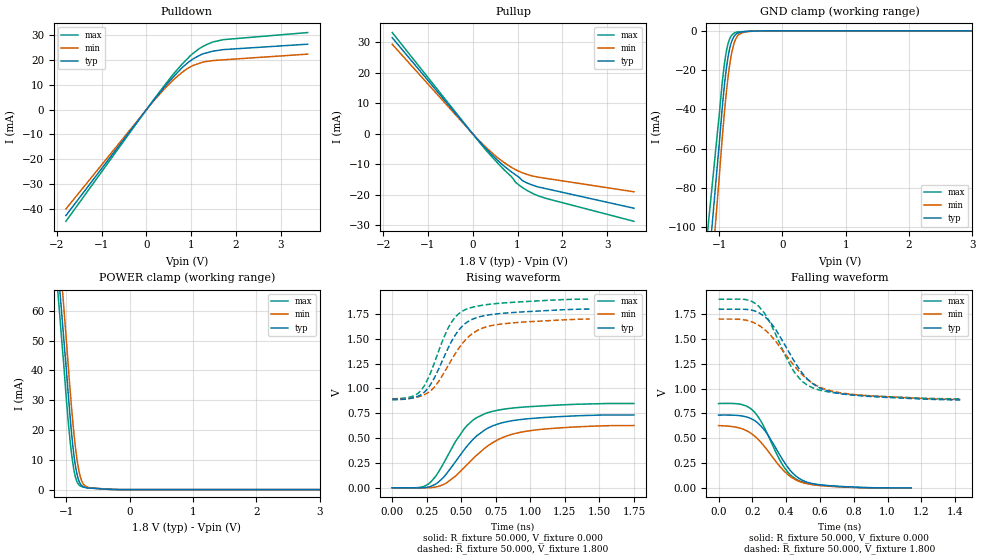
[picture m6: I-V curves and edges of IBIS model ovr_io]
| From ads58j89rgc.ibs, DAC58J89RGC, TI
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[Model]   ovr_io
Model_type I/O
Vinl=4.000E-01
Vinh=1.200E+00
Vref=0.000E+00
Rref=1.000E+06
Cref=0.000E+00
Vmeas=9.000E-01
C_comp   4.650E-13   4.580E-13   4.720E-13
[Voltage Range]   1.800E+00   1.700E+00   1.900E+00
[POWER Clamp Reference]   1.800E+00   1.700E+00   1.900E+00
[GND Clamp Reference]   0.000E+00   0.000E+00   0.000E+00
[Pullup Reference]   1.800E+00   1.700E+00   1.900E+00
[Pulldown Reference]   0.000E+00   0.000E+00   0.000E+00
[Temperature Range]   25   85   -40
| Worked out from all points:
|   slope of the pulldown table from 0 to 0.27 V, typ, clamps not added: 43.7 ohm
|   slope of the pullup table from 0 to 0.27 V, typ, clamps not added: 61.1 ohm
|   GND clamp passes 1 mA (typ) near -0.69 V on its own axis
|   POWER clamp passes 1 mA (typ) near -0.74 V on its own axis
|   rising waveform, R_fixture 50.000, V_fixture 0.000: 20-80 % time 279ps typ, 328ps min, 244ps max; typ from 0 V to 0.733 V
|   falling waveform, R_fixture 50.000, V_fixture 0.000: 20-80 % time 171ps typ, 190ps min, 157ps max; typ from 0.733 V to 0 V
|   rising waveform, R_fixture 50.000, V_fixture 1.800: 20-80 % time 211ps typ, 240ps min, 187ps max; typ from 0.886 V to 1.8 V
|   falling waveform, R_fixture 50.000, V_fixture 1.800: 20-80 % time 215ps typ, 252ps min, 188ps max; typ from 1.8 V to 0.886 V
[GND Clamp]
-1.8V     -354.1mA   -399.6mA   -302.9mA
-1.02V    -65.36mA   -83.09mA   -49.52mA
-940mV    -35.47mA   -50.4mA    -23.16mA
-900mV    -22.91mA   -35.9mA    -13.13mA
-880mV    -17.79mA   -29.53mA   -9.453mA
-840mV    -9.982mA   -18.84mA   -4.57mA
-800mV    -5.195mA   -10.99mA   -2.195mA
-760mV    -2.645mA   -5.947mA   -1.113mA
-720mV    -1.407mA   -3.122mA   -633.1uA
-680mV    -844.7uA   -1.709mA   -465.5uA
-500mV    -201.7uA   -266.4uA   -173.2uA
3.6V      0A         0A         0A
[Power Clamp]
-1.8V     248mA      271.4mA    242.7mA
-1.06V    55.13mA    66.12mA    46.11mA
-1.04V    49.92mA    60.57mA    41.11mA
-980mV    34.21mA    43.87mA    24.61mA
-920mV    18.95mA    27.51mA    12.06mA
-860mV    8.139mA    14.42mA    4.305mA
-820mV    3.987mA    8.204mA    2.055mA
-780mV    1.904mA    4.203mA    1.213mA
-740mV    1.031mA    2.076mA    899.5uA
-680mV    598.2uA    960.3uA    681.9uA
-320mV    65.56uA    63.12uA    153.9uA
3.6V      0A         0A         0A
[Pullup]
-1.8V     31.55mA    29.41mA    33.25mA
140mV     -2.374mA   -2.165mA   -2.578mA
560mV     -8.738mA   -7.85mA    -9.628mA
840mV     -12.2mA    -10.77mA   -13.69mA
960mV     -13.46mA   -11.77mA   -15.92mA
1.04V     -14.3mA    -12.33mA   -16.86mA
1.12V     -15.43mA   -12.81mA   -17.71mA
1.22V     -16.15mA   -13.33mA   -18.62mA
1.44V     -17.33mA   -14.13mA   -20.18mA
1.64V     -17.98mA   -14.59mA   -21.17mA
3.6V      -24.38mA   -18.98mA   -28.67mA
[Pulldown]
-1.8V     -42.6mA    -39.94mA   -44.9mA
160mV     3.747mA    3.477mA    3.981mA
600mV     13.17mA    11.96mA    14.22mA
820mV     17.21mA    15.31mA    18.74mA
1.04V     20.33mA    17.7mA     22.59mA
1.24V     22.25mA    18.93mA    25.14mA
1.34V     22.77mA    19.33mA    26.09mA
1.48V     23.45mA    19.67mA    27.13mA
1.72V     24.1mA     19.99mA    28.1mA
3.6V      26.27mA    22.28mA    30.95mA
[Rising Waveform]
R_fixture = 50.000
V_fixture = 0.000
V_fixture_min = 0.000
V_fixture_max = 0.000
|  time   V(typ)   V(min)   V(max)
0s        0V         0V         0V
200ps     -749.6uV   -635.1uV   4.14mV
270ps     10.41mV    572uV      47.13mV
370ps     104mV      32.31mV    241.9mV
520ps     381.3mV    201.9mV    591.7mV
590ps     494.4mV    299.8mV    686.2mV
680ps     591mV      409.4mV    750.6mV
810ps     659.4mV    512.1mV    792mV
980ps     694.4mV    571.4mV    815.8mV
1.75ns    733.3mV    626.7mV    848.9mV
[Falling Waveform]
R_fixture = 50.000
V_fixture = 0.000
V_fixture_min = 0.000
V_fixture_max = 0.000
|  time   V(typ)   V(min)   V(max)
0s        733.3mV    626.7mV    848.9mV
130ps     726.2mV    600mV      842mV
200ps     691mV      539.7mV    784.3mV
230ps     656.8mV    495.6mV    726.5mV
280ps     562.4mV    398.5mV    577mV
390ps     254.7mV    165.4mV    203mV
430ps     164.7mV    108.1mV    123.3mV
480ps     91.73mV    62.99mV    68.72mV
650ps     22.89mV    16.49mV    20.74mV
1.14ns    0V         0V         0V
[Rising Waveform]
R_fixture = 50.000
V_fixture = 1.800
V_fixture_min = 1.700
V_fixture_max = 1.900
|  time   V(typ)   V(min)   V(max)
0s        885.6mV    891.1mV    896.6mV
140ps     902.2mV    902.4mV    918mV
210ps     939.5mV    925.3mV    983.5mV
300ps     1.094V     1.006V     1.238V
410ps     1.422V     1.243V     1.622V
460ps     1.546V     1.359V     1.724V
520ps     1.644V     1.474V     1.788V
610ps     1.713V     1.58V      1.828V
740ps     1.748V     1.639V     1.854V
1.43ns    1.8V       1.7V       1.9V
[Falling Waveform]
R_fixture = 50.000
V_fixture = 1.800
V_fixture_min = 1.700
V_fixture_max = 1.900
|  time   V(typ)   V(min)   V(max)
0s        1.8V       1.7V       1.9V
160ps     1.798V     1.69V      1.897V
240ps     1.763V     1.636V     1.825V
320ps     1.639V     1.513V     1.611V
440ps     1.297V     1.246V     1.188V
500ps     1.146V     1.131V     1.067V
560ps     1.046V     1.051V     1.006V
650ps     974.5mV    984.4mV    967mV
790ps     935mV      942.7mV    939.1mV
1.43ns    885.6mV    891.1mV    896.6mV
[Ramp]
dV/dt_r   4.3961E-01/2.7828E-10   3.7604E-01/3.2723E-10   5.0831E-01/2.4320E-10
dV/dt_f   5.4865E-01/2.1387E-10   4.8537E-01/2.5127E-10   6.0206E-01/1.8780E-10
R_load = 50
